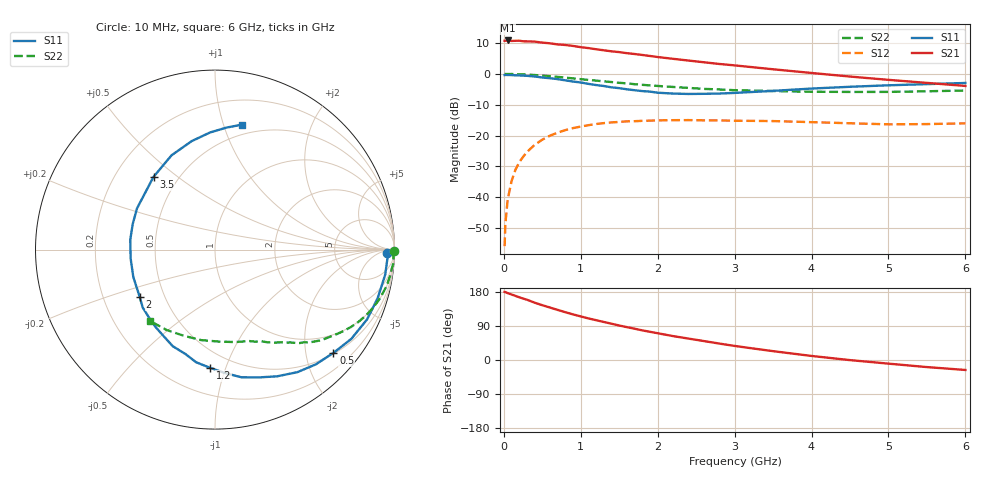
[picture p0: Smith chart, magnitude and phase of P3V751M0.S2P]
! SIEMENS Small Signal Semiconductors
! BFP181
! Si NPN RF Bipolar Junction Transistor in SOT143
! VCE = 0.75 V  IC = 1 mA
! Common Emitter S-Parameters:  March  1996
# GHz  S  MA  R  50
!  f  S11  S21  S12  S22
! GHz  MAG  ANG  MAG  ANG  MAG  ANG  MAG  ANG
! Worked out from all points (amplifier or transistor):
!   36 points, 10 MHz to 6 GHz, reference 50 ohm
!   highest |S21| = 10.9 dB at 50 MHz (marker M1)
!   |S21| within 3 dB of that: start of sweep to 1.242 GHz
!   unconditionally stable (mu >= 1): 2.83 GHz to end of sweep
!   at 250 MHz: K = 0.10, MSG = 18.8 dB, |S12| = -26.9 dB
!   at 1.4 GHz: K = 0.54, MSG = 11.5 dB, |S12| = -15.7 dB
!   at 6 GHz: K = 1.43, MAG = 2.2 dB, |S12| = -16.0 dB
!   S11 on the Smith chart (normalised r, x): 10 MHz: 41, -18; 500 MHz: 0.52, -2.58; 1.2 GHz: 0.38, -0.89; 2 GHz: 0.36, -0.25; 3.5 GHz: 0.37, +0.41; 6 GHz: 0.41, +1.16
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0.01  0.9599 -1.0  3.45 179.6  0.0016 88.7  0.9984 -0.4
0.02  0.9628 -2.0  3.449 179.2  0.0037 90.0  0.998 -0.8
0.05  0.9607 -3.9  3.492 176.5  0.0092 89.5  0.9948 -2.0
0.1  0.9585 -8.4  3.429 172.9  0.0181 82.8  0.9973 -4.1
0.2  0.9457 -16.6  3.461 165.6  0.0367 79.0  0.9866 -8.4
0.4  0.908 -33.2  3.344 151.3  0.0704 68.3  0.9595 -16.3
0.5  0.8755 -41.1  3.224 144.6  0.0857 62.9  0.9395 -20.0
0.6  0.8511 -48.7  3.138 138.4  0.0995 58.2  0.9184 -23.5
0.8  0.7862 -63.9  2.949 126.1  0.1225 49.2  0.8712 -29.7
0.9  0.752 -71.3  2.845 120.3  0.132 44.9  0.8455 -32.6
1.1  0.6891 -85.6  2.627 109.7  0.1473 37.5  0.7985 -37.8
1.2  0.6594 -92.3  2.512 105.0  0.1538 33.7  0.7785 -40.4
1.6  0.5629 -120.0  2.17 86.7  0.1699 23.0  0.7026 -47.8
1.8  0.5262 -134.9  2.031 78.2  0.173 18.8  0.6655 -51.0
2  0.4954 -147.9  1.88 70.6  0.1761 14.6  0.638 -54.1
2.2  0.48 -161.5  1.758 63.1  0.1775 10.7  0.6142 -57.5
2.8  0.48 162.8  1.451 43.4  0.1761 2.4  0.5597 -66.4
3.5  0.5307 130.2  1.189 23.3  0.1716 -4.3  0.5273 -77.7
4  0.5786 114.7  1.036 10.7  0.1649 -7.6  0.5129 -87.6
4.5  0.6183 102.1  0.906 -0.3  0.1581 -9.9  0.5102 -98.6
5.5  0.6828 84.6  0.715 -18.7  0.1534 -8.1  0.5226 -120.9
6  0.7129 77.7  0.638 -26.3  0.1576 -7.4  0.5377 -132.3
